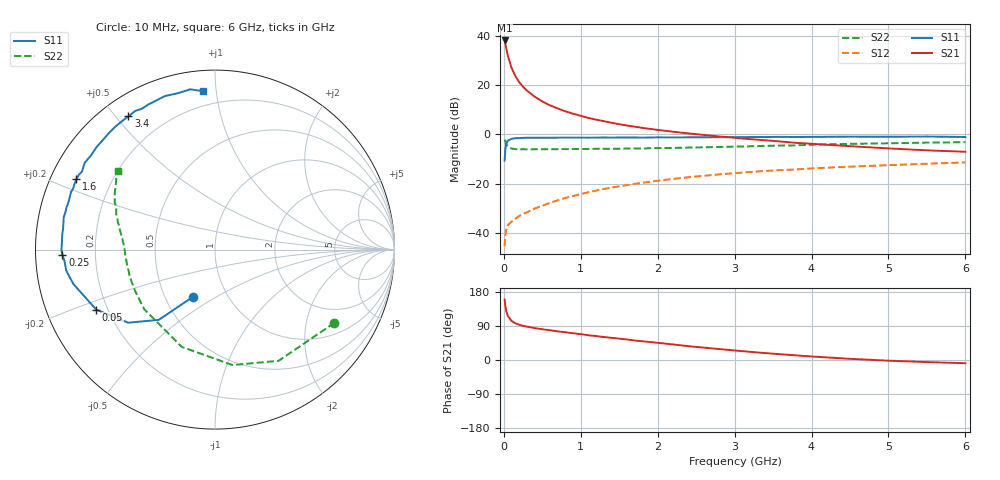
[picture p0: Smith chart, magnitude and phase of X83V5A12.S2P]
! SIEMENS Small Signal Semiconductors
! BFP136W
! Si NPN RF Bipolar Junction Transistor in SOT343
! VCE = 3.5 V  IC = 120 mA
! Common Emitter S-Parameters:  September  1994
# GHz  S  MA  R  50
!  f  S11  S21  S12  S22
! GHz  MAG  ANG  MAG  ANG  MAG  ANG  MAG  ANG
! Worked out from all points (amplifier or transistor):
!   40 points, 10 MHz to 6 GHz, reference 50 ohm
!   highest |S21| = 38.3 dB at 10 MHz (marker M1)
!   |S21| within 3 dB of that: start of sweep to 30.31 MHz
!   unconditionally stable (mu >= 1): 499.6 MHz to 2.95 GHz
!   at 200 MHz: K = 0.72, MSG = 27.2 dB, |S12| = -33.2 dB
!   at 1.5 GHz: K = 1.10, MAG = 10.7 dB, |S12| = -21.1 dB
!   at 6 GHz: K = 0.98, MSG = 2.2 dB, |S12| = -11.4 dB
!   S11 on the Smith chart (normalised r, x): 10 MHz: 0.68, -0.40; 50 MHz: 0.16, -0.23; 250 MHz: 0.08, -0.02; 1.6 GHz: 0.08, +0.24; 3.4 GHz: 0.08, +0.54; 6 GHz: 0.11, +0.92
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0.01  0.2927 -115.3  81.84 159.6  0.0053 68.7  0.7806 -31.5
0.02  0.5016 -128.7  69.8 142.7  0.009 56.6  0.7138 -60.2
0.03  0.6323 -139.9  58.25 131.0  0.0114 49.2  0.6509 -81.3
0.05  0.7415 -153.2  41.23 117.1  0.0142 39.8  0.5728 -108.9
0.1  0.8123 -166.4  22.65 103.0  0.0167 38.4  0.5156 -139.9
0.15  0.8372 -172.0  15.38 96.8  0.0192 40.9  0.5012 -152.5
0.2  0.8404 -175.4  11.56 93.0  0.0218 43.5  0.4977 -159.3
0.25  0.8506 -178.1  9.336 90.1  0.024 46.4  0.4973 -163.7
0.3  0.8552 -179.7  7.804 88.1  0.0259 48.6  0.4957 -166.6
0.4  0.8542 176.7  5.879 84.2  0.0309 53.0  0.4972 -170.6
0.5  0.8551 174.1  4.688 81.1  0.0352 55.5  0.4979 -173.3
0.6  0.8544 172.2  3.91 78.6  0.0405 57.8  0.499 -175.1
0.7  0.8578 169.8  3.374 75.6  0.0455 59.4  0.5005 -176.4
0.9  0.8591 166.1  2.639 70.6  0.0556 60.6  0.5024 -179.1
1.1  0.8582 161.8  2.159 65.2  0.0664 61.2  0.5059 179.3
1.6  0.8662 153.0  1.518 54.2  0.0928 59.6  0.5151 175.3
2.2  0.8675 142.9  1.133 41.0  0.124 55.3  0.5301 170.7
3.2  0.8834 126.1  0.8 21.6  0.1712 45.7  0.5723 161.9
3.4  0.8852 123.0  0.759 18.2  0.1807 43.5  0.585 160.2
4.5  0.8996 108.1  0.575 3.1  0.2204 33.4  0.6412 150.6
5.5  0.9038 98.8  0.474 -5.5  0.2528 25.6  0.6797 144.0
6  0.8856 94.5  0.443 -8.5  0.269 21.2  0.6943 141.1
